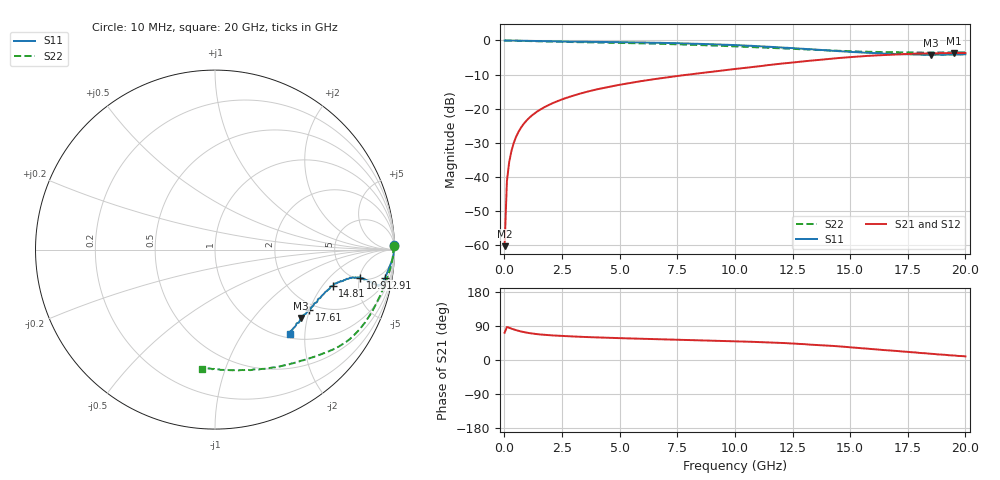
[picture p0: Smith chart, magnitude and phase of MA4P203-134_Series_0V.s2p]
! AWR Design Environment (9226) Thu Aug 19 14:29:25 2021
! Document = '0V'
! nPorts: 2, nXvals: 201
# GHz S DB R 50
!Freq DBS11 AngS11 DBS21 AngS21 DBS12 AngS12 DBS22 AngS22
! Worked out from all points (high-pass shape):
!   201 points, 10 MHz to 20 GHz, reference 50 ohm
!   highest |S21| = -3.68 dB at 19.51 GHz (marker M1); lowest = -60.2 dB at 10 MHz (marker M2)
!   |S21| within 3 dB of the highest: 12.19 GHz to end of sweep
!   lowest |S11| = -4.3 dB at 18.51 GHz (marker M3), VSWR 4.16, Z = 75.3 - j91.6 ohm
!   |S11| at or under -10 dB: nowhere
!   |S22| runs from -3.6 to 0.0 dB; largest |S21 - S12| = 0.022
!   S11 on the Smith chart (normalised r, x): 10 MHz: 16, +83; 2.91 GHz: 3, -12; 10.91 GHz: 5.27, -5.18; 14.81 GHz: 3.32, -2.54; 17.61 GHz: 1.81, -1.99; 20 GHz: 1.08, -1.67
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0.01  -0.04 1.3  -60.21 72.0  -60.73 53.0  -0.02 1.2
0.11  -0.04 -0.6  -41.17 87.1  -41.01 86.8  -0.06 -0.9
0.21  -0.04 -1.1  -35.54 85.1  -35.53 84.9  -0.07 -1.8
0.31  -0.05 -1.6  -32.26 82.6  -32.27 82.8  -0.08 -2.6
0.41  -0.06 -2.0  -29.93 80.6  -29.96 80.8  -0.09 -3.5
0.51  -0.07 -2.5  -28.19 78.7  -28.21 79.0  -0.11 -4.2
0.81  -0.11 -3.7  -24.68 74.1  -24.68 74.3  -0.17 -6.5
1.31  -0.19 -5.3  -21.36 69.1  -21.36 69.3  -0.26 -10.0
2.01  -0.27 -7.3  -18.63 65.2  -18.63 65.5  -0.37 -14.4
2.91  -0.35 -9.3  -16.33 62.3  -16.32 62.8  -0.49 -19.4
3.41  -0.39 -10.2  -15.34 61.0  -15.33 61.6  -0.54 -22.0
4.71  -0.49 -11.7  -13.35 58.3  -13.35 58.9  -0.70 -28.0
6.71  -0.69 -12.4  -11.16 54.9  -11.14 56.0  -0.99 -35.3
10.01  -1.36 -11.3  -8.37 49.5  -8.32 51.2  -1.75 -46.6
10.91  -1.67 -10.9  -7.68 47.8  -7.58 49.4  -2.01 -50.5
13.41  -2.64 -13.3  -5.84 40.3  -5.75 41.7  -2.75 -64.7
14.81  -3.27 -17.2  -5.00 34.6  -4.91 35.8  -3.11 -73.8
16.71  -3.89 -26.8  -4.22 25.1  -4.18 26.7  -3.44 -85.6
17.61  -4.09 -32.6  -3.92 20.7  -3.92 22.4  -3.50 -89.8
18.51  -4.26 -38.4  -3.80 16.4  -3.82 17.7  -3.57 -92.9
19.51  -4.16 -45.4  -3.68 11.9  -3.73 13.4  -3.53 -95.8
20  -4.07 -48.4  -3.69 9.4  -3.78 11.3  -3.49 -96.3
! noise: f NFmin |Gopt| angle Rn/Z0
0.01  0  1  0  2e-20
2.21  0  1  0  2e-20
4.41  0  1  0  2e-20
6.61  0  1  0  2e-20
8.81  0  1  0  2e-20
11.11  0  1  0  2e-20
13.31  0  1  0  2e-20
15.51  0  1  0  2e-20
17.71  0  1  0  2e-20
20  0  1  0  2e-20
